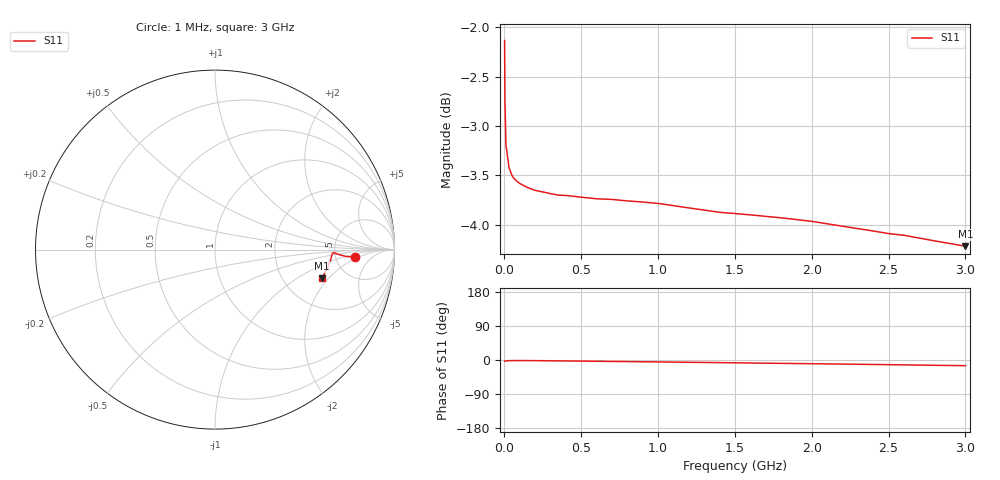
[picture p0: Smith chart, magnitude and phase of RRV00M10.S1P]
! SIEMENS Small Signal Semiconductors
! BA595
! Si PIN Diode in SOD323
! IF = 0.1 mA
! S-Parameters:  July  1992
# GHz  S  MA  R  50
!  f  S11
! GHz  MAG  ANG
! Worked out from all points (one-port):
!   33 points, 1 MHz to 3 GHz, reference 50 ohm
!   lowest |S11| = -4.2 dB at 3 GHz (marker M1), VSWR 4.20, Z = 164 - j83.8 ohm
!   |S11| at or under -10 dB: nowhere
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0.001  0.7822 -3.1
0.003  0.73 -3.0
0.01  0.6921 -2.3
0.03  0.6741 -1.8
0.05  0.6679 -1.6
0.06  0.6661 -1.6
0.08  0.6637 -1.6
0.1  0.6619 -1.5
0.15  0.6588 -1.6
0.2  0.6566 -1.7
0.3  0.6541 -2.1
0.35  0.653 -2.3
0.4  0.6527 -2.5
0.5  0.6514 -2.9
0.6  0.6502 -3.4
0.8  0.6486 -4.2
0.9  0.6477 -4.7
1  0.6467 -5.1
1.2  0.6433 -6.0
1.4  0.64 -6.9
1.6  0.6381 -7.9
1.8  0.6359 -8.9
2  0.6333 -9.8
2.4  0.6262 -11.8
2.5  0.6243 -12.3
2.6  0.6231 -12.9
2.8  0.619 -14.0
3  0.6152 -15.0
